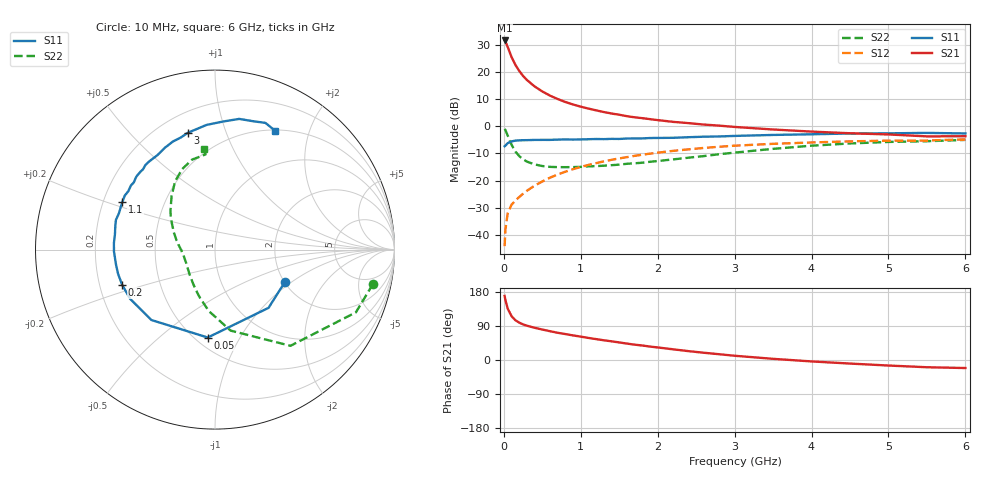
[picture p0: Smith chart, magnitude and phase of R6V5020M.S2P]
! SIEMENS Small Signal Semiconductors
! BFR193
! Si NPN RF Bipolar Junction Transistor in SOT23
! VCE = 0.5 V  IC = 20 mA
! Common Emitter S-Parameters:  May  1996
# GHz  S  MA  R  50
!  f  S11  S21  S12  S22
! GHz  MAG  ANG  MAG  ANG  MAG  ANG  MAG  ANG
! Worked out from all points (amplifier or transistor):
!   36 points, 10 MHz to 6 GHz, reference 50 ohm
!   highest |S21| = 31.8 dB at 10 MHz (marker M1)
!   |S21| within 3 dB of that: start of sweep to 58.02 MHz
!   unconditionally stable (mu >= 1): 432.5 MHz to 2.658 GHz; 5.433 GHz to end of sweep
!   at 250 MHz: K = 0.87, MSG = 21.8 dB, |S12| = -24.9 dB
!   at 1.4 GHz: K = 1.05, MAG = 7.2 dB, |S12| = -12.4 dB
!   at 6 GHz: K = 1.00, MAG = 0.2 dB, |S12| = -4.8 dB
!   S11 on the Smith chart (normalised r, x): 10 MHz: 2.03, -0.89; 50 MHz: 0.57, -0.74; 200 MHz: 0.30, -0.17; 1.1 GHz: 0.28, +0.22; 3 GHz: 0.32, +0.74; 6 GHz: 0.51, +1.50
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0.01  0.4298 -24.5  38.95 169.2  0.0061 78.9  0.9006 -12.3
0.02  0.4408 -47.4  37.46 158.8  0.0123 73.9  0.8593 -24.0
0.05  0.4915 -94.7  29.52 135.8  0.0247 60.3  0.6812 -51.9
0.1  0.5287 -132.1  19.31 115.7  0.0357 53.9  0.4596 -79.1
0.15  0.5468 -149.9  13.76 104.9  0.0426 54.2  0.3449 -95.6
0.2  0.5534 -159.3  10.65 98.7  0.0495 56.4  0.283 -107.0
0.25  0.5567 -166.0  8.606 93.9  0.0569 58.5  0.2462 -116.2
0.3  0.5578 -171.2  7.226 90.5  0.0645 60.2  0.2238 -123.4
0.4  0.5631 -179.0  5.5 85.0  0.0803 62.4  0.1983 -135.5
0.5  0.5643 176.2  4.437 80.4  0.096 63.8  0.1852 -144.7
0.6  0.5641 171.1  3.719 76.0  0.1128 63.9  0.1788 -151.0
0.7  0.5706 166.8  3.215 71.8  0.1291 63.7  0.1768 -156.5
0.9  0.5721 159.4  2.545 64.9  0.1623 62.0  0.177 -166.5
1.1  0.5805 152.7  2.139 58.2  0.1944 59.6  0.1825 -172.6
1.3  0.5824 146.0  1.848 52.0  0.2259 56.9  0.1877 -179.1
1.6  0.5976 137.3  1.547 43.3  0.2709 52.3  0.2039 172.9
2.2  0.6164 121.3  1.216 28.2  0.3536 42.4  0.2457 158.2
3  0.6679 103.2  0.979 11.2  0.4406 28.8  0.328 139.2
3.5  0.6963 93.9  0.878 3.1  0.477 20.7  0.385 128.9
4.5  0.7406 79.5  0.748 -9.4  0.5297 7.0  0.4847 112.1
5.5  0.7598 68.3  0.655 -19.1  0.5481 -5.6  0.5332 95.6
6  0.7422 63.2  0.66 -21.2  0.5773 -9.4  0.5634 96.5
